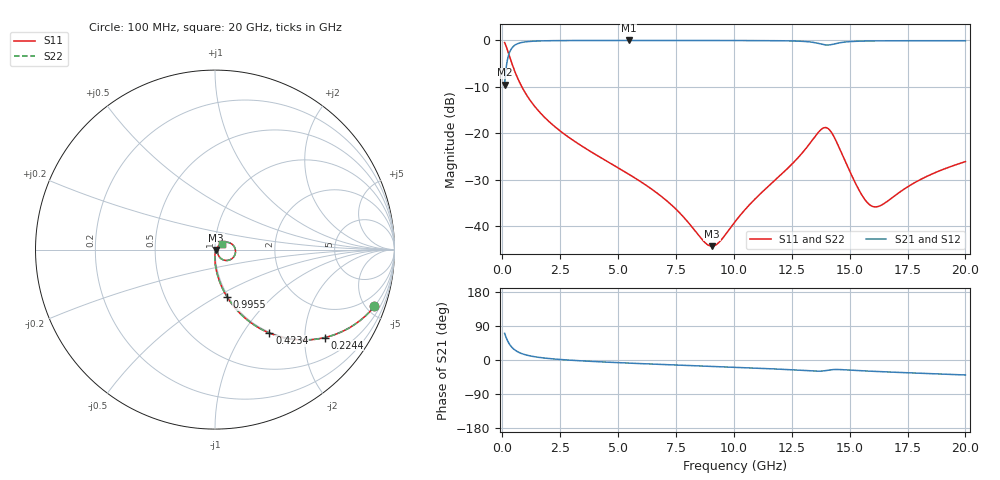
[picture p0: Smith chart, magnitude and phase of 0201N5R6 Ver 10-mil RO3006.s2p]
# GHz S MA R 50
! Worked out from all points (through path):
!   1601 points, 100 MHz to 20 GHz, reference 50 ohm
!   highest |S21| = -0.04 dB at 5.461 GHz (marker M1); lowest = -9.6 dB at 100 MHz (marker M2)
!   group delay of S21, straight-line fit = 7.43 ps
!   lowest |S11| = -44.3 dB at 9.055 GHz (marker M3), VSWR 1.01, Z = 50.6 - j0.218 ohm
!   |S11| at or under -10 dB: 842.8 MHz to end of sweep
!   |S22| runs from -44.3 to -0.5 dB; largest |S21 - S12| = 0
!   S11 on the Smith chart (normalised r, x): 100 MHz: 0.99, -5.61; 224.4 MHz: 0.99, -2.50; 423.4 MHz: 0.99, -1.32; 995.5 MHz: 0.99, -0.56; 20 GHz: 1.08, +0.07
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0.1  0.9428 -19.6  0.3328 70.3  0.3328 70.3  0.9428 -19.6
0.224375  0.7832 -38.8  0.6205 51.1  0.6205 51.1  0.7832 -38.8
0.423375  0.5548 -56.9  0.8304 32.9  0.8304 32.9  0.5548 -56.9
0.64725  0.3991 -67.5  0.9152 22.3  0.9152 22.3  0.3991 -67.5
0.9955  0.2709 -75.8  0.9607 13.8  0.9607 13.8  0.2709 -75.8
1.953188  0.1382 -84.7  0.9878 4.3  0.9878 4.3  0.1382 -84.7
3.420812  0.07315 -89.6  0.9938 -2.3  0.9938 -2.3  0.07315 -89.6
5.460562  0.03629 -91.3  0.9948 -8.2  0.9948 -8.2  0.03629 -91.3
6.741625  0.02217 -88.6  0.9947 -11.4  0.9947 -11.4  0.02217 -88.6
8.731625  0.006743 -45.3  0.9939 -16.2  0.9939 -16.2  0.006743 -45.3
9.055  0.006102 -20.7  0.9937 -16.9  0.9937 -16.9  0.006102 -20.7
9.390812  0.006836 4.8  0.9934 -17.7  0.9934 -17.7  0.006836 4.8
10.05  0.01116 32.8  0.9928 -19.3  0.9928 -19.3  0.01116 32.8
13.37081  0.08307 29.0  0.9531 -28.9  0.9531 -28.9  0.08307 29.0
13.80612  0.1116 3.7  0.9041 -29.1  0.9041 -29.1  0.1116 3.7
14.07975  0.1118 -21.3  0.8883 -26.8  0.8883 -26.8  0.1118 -21.3
14.7265  0.05555 -57.6  0.9521 -25.7  0.9521 -25.7  0.05555 -57.6
15.7215  0.01846 -36.1  0.9813 -29.0  0.9813 -29.0  0.01846 -36.1
16.13194  0.01614 -10.4  0.9844 -30.2  0.9844 -30.2  0.01614 -10.4
16.69162  0.01902 15.6  0.9866 -31.7  0.9866 -31.7  0.01902 15.6
18.14681  0.03261 35.5  0.9883 -35.2  0.9883 -35.2  0.03261 35.5
20  0.04954 38.6  0.9882 -39.5  0.9882 -39.5  0.04954 38.6
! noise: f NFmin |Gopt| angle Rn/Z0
0.1  0.0009029  0.9522  0.3844  0.004244
2.301  0.00503  0.8155  4.477  0.00569
4.515  0.008366  0.7863  8.581  0.008006
6.729  0.0114  0.7692  12.68  0.009942
8.943  0.01453  0.7613  16.76  0.01208
11.14  0.01913  0.7737  20.78  0.01671
13.36  0.04792  0.8855  24.83  0.08669
15.57  0.03475  0.8233  28.87  0.03874
17.79  0.02747  0.756  32.76  0.02098
20  0.02793  0.7354  36.59  0.01906
